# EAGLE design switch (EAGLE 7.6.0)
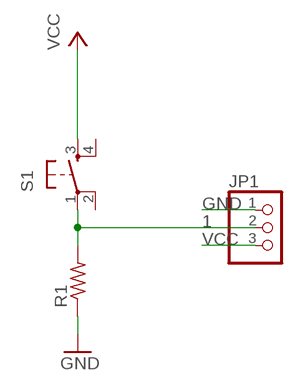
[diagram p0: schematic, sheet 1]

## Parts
JP1  PINHD-1X3/90  [1X03/90]
R1  RES-US1206FAB  [R1206FAB]
S1  6MM_SWITCH6MM_SWITCH  [6MM_SWITCH]

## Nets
1: JP1.2 R1.2 S1.1(P)
GND: JP1.1 R1.1
VCC: JP1.3 S1.3(S)
Unconnected: S1.2(P1) S1.4(S1)

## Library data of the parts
JP1 = pinhead:PINHD-1X3: PIN HEADER
R1 = fab:RES-US: Resistor (US Symbol)
S1 = fab:6MM_SWITCH: OMRON SWITCH

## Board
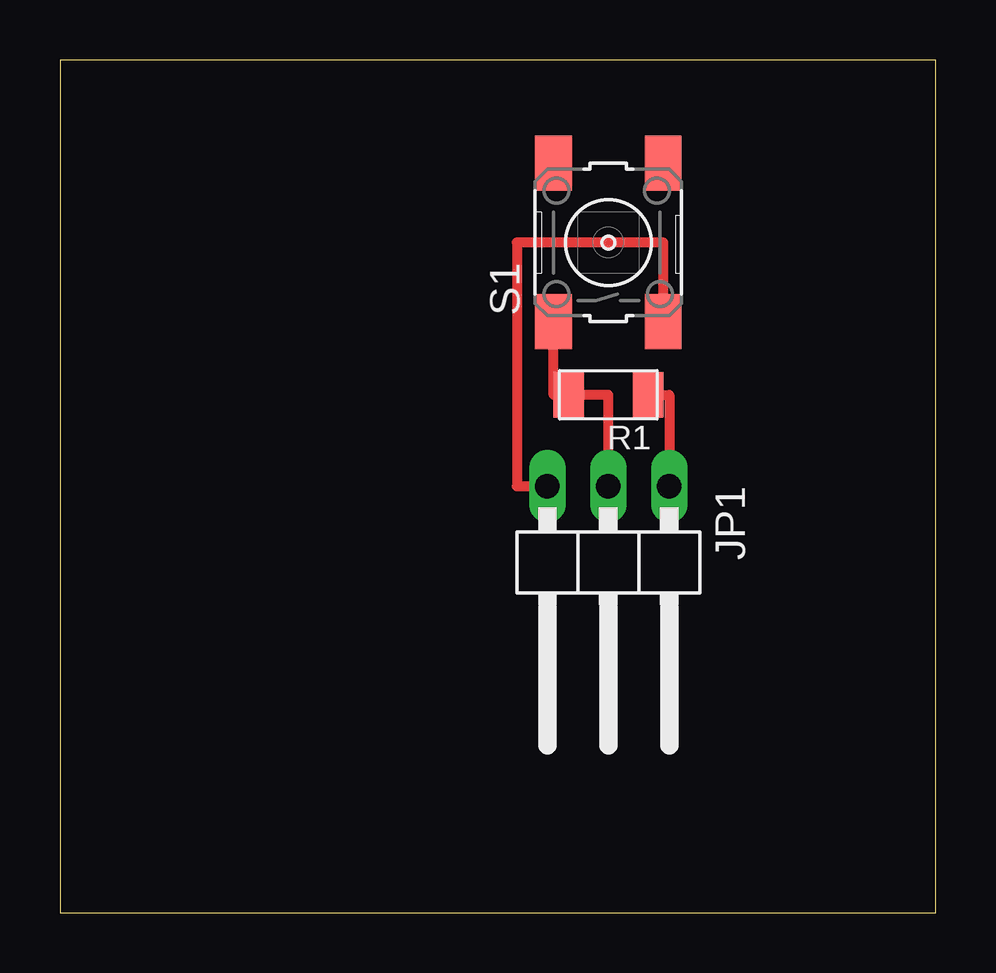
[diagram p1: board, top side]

Size 36.5 x 35.55 mm. Coordinates in mm from the lower left corner, seen from the top.
Outline: 0,0 36.5,0 36.5,35.55 0,35.55 0,0
Copper layers (1*16): Top 0.035mm / dielectric 1.5mm / Bottom 0.035mm
Design rules "default": minimum track width 10mil, minimum drill 24mil, track to track 8mil, track to pad 8mil, pad to pad 8mil, via to via 8mil, smd to smd 8mil, copper to edge 40mil, drill to drill 8mil, minimum pad ring 10mil, minimum via ring 8mil, stop-mask expansion 4mil, vias tented up to drill 0mil, thermal gap 10mil

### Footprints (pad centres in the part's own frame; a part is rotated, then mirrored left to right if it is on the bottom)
1X03/90 = drill 1.016 long: 1 -2.54,-3.81; 2 0,-3.81; 3 2.54,-3.81
R1206FAB = smd 1.27 x 1.905: 1 -1.651,0; 2 1.651,0
6MM_SWITCH = smd 2.286 x 1.524: 1 -3.302,2.286; 2 3.302,2.286; 3 -3.302,-2.286; 4 3.302,-2.286

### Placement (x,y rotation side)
JP1  22.86,13.97 180 top
R1  22.86,21.59 180 top
S1  22.86,27.94 90 top

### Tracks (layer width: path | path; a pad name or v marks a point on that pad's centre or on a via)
1
  Top 0.406: JP1.2 22.86,21.59 R1.2 20.57,21.59 S1.1
GND
  Top 0.406: R1.1 25.4,21.59 JP1.1
VCC
  Top 0.406: S1.3 25.15,27.94 19.05,27.94 19.05,17.78 JP1.3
